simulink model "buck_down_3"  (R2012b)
settings: Solver=ode45  StartTime=0.0  StopTime=10.0  RelTol=1e-3
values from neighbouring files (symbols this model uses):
  alpha = 1/(1+Rc/R)    (= 0.909090909091)    [buck_down3.m]    (also in unwucht_4.m = 2*pi*(fmax-fmin)/T1,)
  C = 100e-6    (= 0.0001)    [boost_up1.m]    (also in buck_boost1.m = 0.0002; buck_boost2.m = 0.0002; buck_down1.m; buck_down2.m)
  f0 = 0.2e5    (= 20000)    [boost_up1.m]    (also in buck_boost1.m; buck_boost2.m; buck_down1.m; buck_down2.m)
  L = 0.001    [boost_up1.m]    (also in buck_boost1.m; buck_boost2.m; buck_down1.m; buck_down2.m)
  R = 5    [boost_up1.m]    (also in buck_boost1.m; buck_boost2.m; buck_down1.m = 2*Rmax,; buck_down2.m = 0.1*Rmax,)
  Rc = 0.5    [buck_down3.m]
  Ui = 5    [boost_up1.m]    (also in buck_boost1.m; buck_boost2.m; buck_down1.m; buck_down2.m)

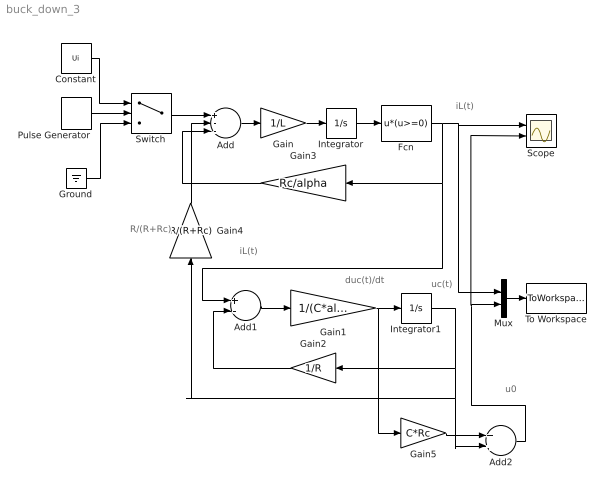
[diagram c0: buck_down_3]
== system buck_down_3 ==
  note: duc(t)/dt
  note: u0
  note: R/(R+Rc)
  note: iL(t)
  note: uc(t)
  note: iL(t)
  Add : Sum  Inputs=+--
  Add1 : Sum  Inputs=+-
  Add2 : Sum
  Constant : Constant  Value=Ui
  Fcn : Fcn  Expr=u*(u>=0)
  Gain : Gain  Gain=1/L
  Gain1 : Gain  Gain=1/(C*alpha)
  Gain2 : Gain  Gain=1/R
  Gain3 : Gain  Gain=Rc/alpha
  Gain4 : Gain  Gain=R/(R+Rc)
  Gain5 : Gain  Gain=C*Rc
  Ground : Ground
  Integrator : Integrator
  Integrator1 : Integrator
  Mux : Mux  Inputs=2
  Pulse Generator : DiscretePulseGenerator  PulseType=Time based  Period=1/f0  PulseWidth=50
  Scope : Scope  NumInputPorts=2
  Switch : Switch  Criteria=u2 > Threshold  Threshold=0.5  ZeroCross=off  SampleTime=0
  To Workspace : ToWorkspace  VariableName=y  SampleTime=-1  SaveFormat=Structure With Time
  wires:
  Pulse Generator/1 -> Switch/2
  Add/1 -> Gain/1
  Gain/1 -> Integrator/1
  Gain1/1 -> Gain5/1, Integrator1/1
  Add1/1 -> Gain1/1
  Gain2/1 -> Add1/2
  Ground/1 -> Switch/3
  Constant/1 -> Switch/1
  Switch/1 -> Add/1
  Integrator1/1 -> Gain2/1, Add2/2, Gain4/1
  Integrator/1 -> Fcn/1
  Fcn/1 -> Gain3/1, Add1/1, Mux/1, Scope/1
  Mux/1 -> To Workspace/1
  Gain3/1 -> Add/3
  Gain4/1 -> Add/2
  Gain5/1 -> Add2/1
  Add2/1 -> Scope/2, Mux/2
